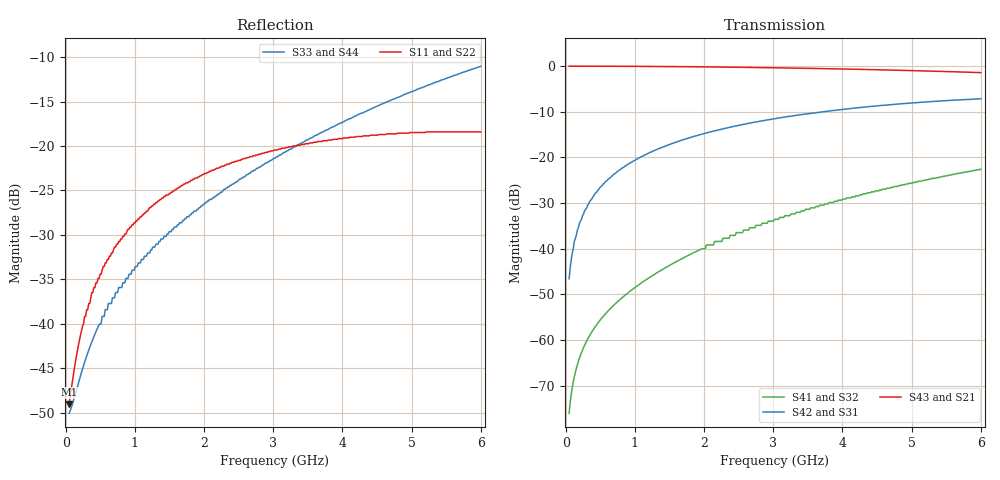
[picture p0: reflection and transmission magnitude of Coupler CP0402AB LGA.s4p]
!	AVX THIN FILM OPERATION
!	CP0402 HIGH DIRECTIVITY COUPLERS
!	P/N CP0402AxxxxBLTR
!	Network	Analyzer HP8720ES.07.64:Feb23,2000 Serial No.US39172382
!	Hewlett-Packard
!	24July2003	02:45:57
# MHZ S MA R 50
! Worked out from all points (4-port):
!   400 points, 50 MHz to 6 GHz, reference 50 ohm
!   strongest paths, dB at 50 MHz, 1.541 GHz, 3.032 GHz, 4.524 GHz, 6 GHz:
!     S43: 0.0, -0.1, -0.4, -0.8, -1.4
!     S21: 0.0, -0.1, -0.4, -0.7, -1.1
!     S42: -46.6, -17.0, -11.5, -8.7, -7.2
!     S31: -46.6, -17.0, -11.5, -8.7, -7.2
!     S41: -76.0, -43.3, -33.6, -27.3, -22.6
!     S32: -76.0, -43.3, -33.6, -27.3, -22.6
!   lowest |S11| = -49.0 dB at 50 MHz (marker M1), VSWR 1.01, Z = 50.3 - j0.193 ohm
!   |S11| at or under -10 dB: start of sweep to end of sweep
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50  0.003534 -32.8  0.997 -0.5  0.00469 89.4  0.0001576 -88.9
    0.997 -0.5  0.003534 -32.8  0.0001576 -88.9  0.00469 89.4
    0.00469 89.4  0.0001576 -88.9  0.003138 17.2  0.997 -0.7
    0.0001576 -88.9  0.00469 89.4  0.997 -0.7  0.003138 17.2
124.561  0.005572 -58.9  0.997 -1.2  0.012 88.5  0.000394 -88.6
         0.997 -1.2  0.005572 -58.9  0.000394 -88.6  0.012 88.5
         0.012 88.5  0.000394 -88.6  0.003828 37.2  0.997 -1.7
         0.000394 -88.6  0.012 88.5  0.997 -1.7  0.003828 37.2
348.246  0.013 -80.7  0.996 -3.5  0.033 85.9  0.001126 -87.7
         0.996 -3.5  0.013 -80.7  0.001126 -87.7  0.033 85.9
         0.033 85.9  0.001126 -87.7  0.007383 61.5  0.996 -4.6
         0.001126 -87.7  0.033 85.9  0.996 -4.6  0.007383 61.5
706.14  0.027 -90.4  0.994 -7.1  0.066 81.8  0.002448 -87.3
        0.994 -7.1  0.027 -90.4  0.002448 -87.3  0.066 81.8
        0.066 81.8  0.002448 -87.3  0.014 68.3  0.995 -9.4
        0.002448 -87.3  0.066 81.8  0.995 -9.4  0.014 68.3
1257.895  0.046 -98.3  0.989 -12.5  0.117 75.4  0.0051 -90.2
          0.989 -12.5  0.046 -98.3  0.0051 -90.2  0.117 75.4
          0.117 75.4  0.0051 -90.2  0.027 65.9  0.99 -16.7
          0.0051 -90.2  0.117 75.4  0.99 -16.7  0.027 65.9
3166.667  0.097 -115.5  0.952 -30.8  0.276 53.6  0.023 -123.2
          0.952 -30.8  0.097 -115.5  0.023 -123.2  0.276 53.6
          0.276 53.6  0.023 -123.2  0.092 42.4  0.953 -42.0
          0.023 -123.2  0.276 53.6  0.953 -42.0  0.092 42.4
6000  0.12 -129.0  0.884 -55.3  0.438 21.6  0.074 169.5
      0.884 -55.3  0.12 -129.0  0.074 169.5  0.438 21.6
      0.438 21.6  0.074 169.5  0.281 3.1  0.847 -80.0
      0.074 169.5  0.438 21.6  0.847 -80.0  0.281 3.1
